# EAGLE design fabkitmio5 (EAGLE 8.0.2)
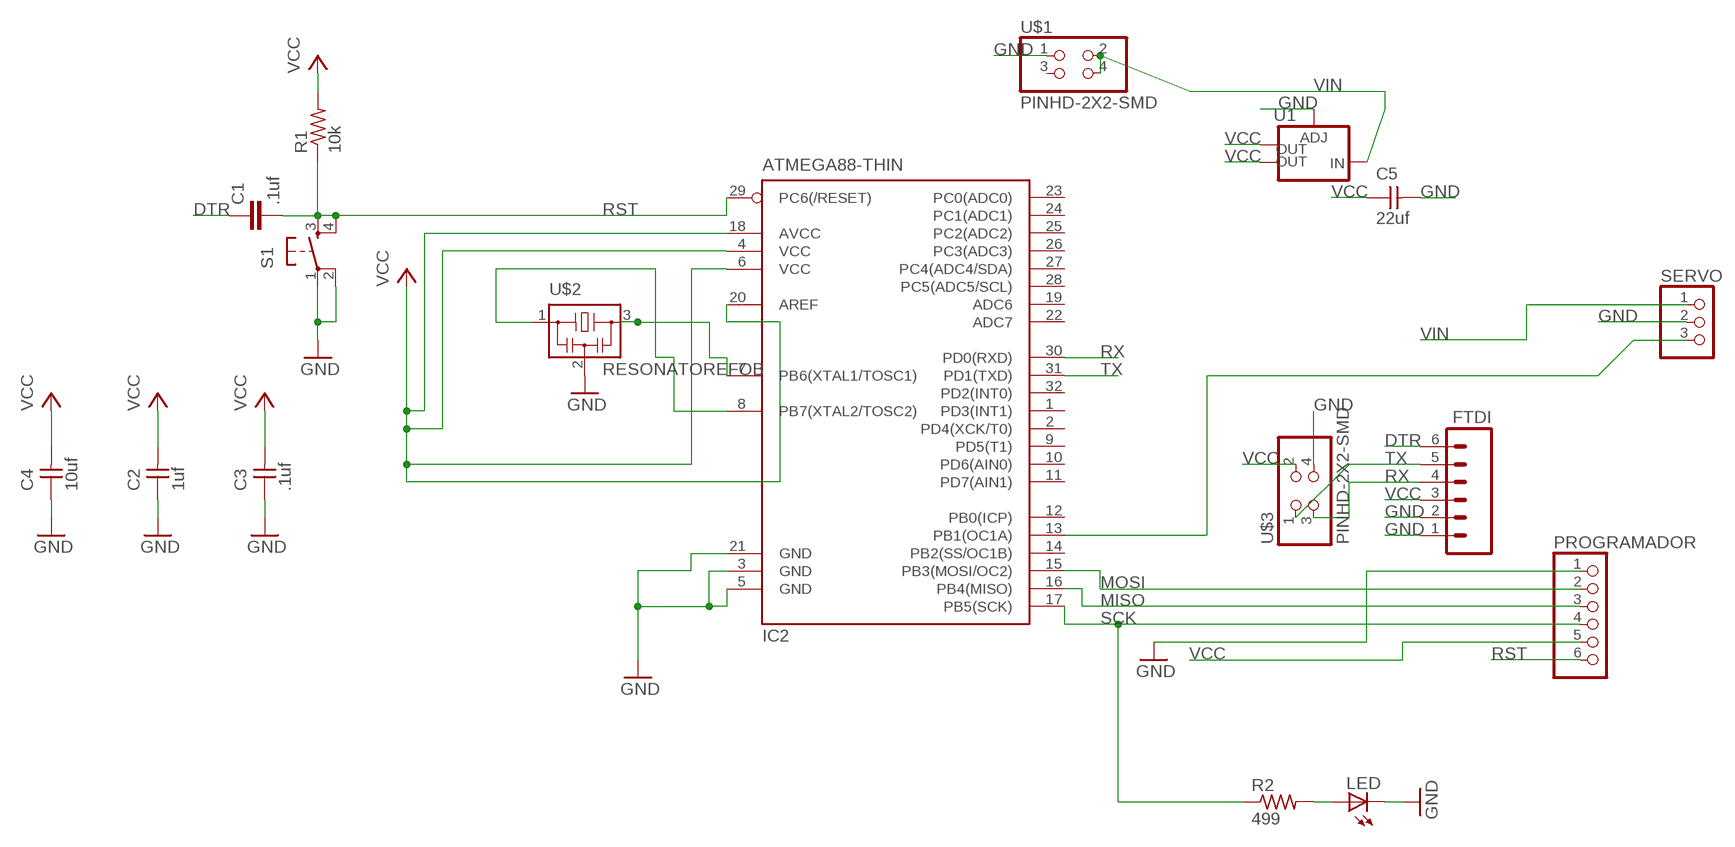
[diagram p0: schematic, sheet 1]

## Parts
C1  .1uf  C-EUC1206  [C1206]
C2  1uf  UNPOLARIZED_CAPACITOR1206  [1206]
C3  .1uf  UNPOLARIZED_CAPACITOR1206  [1206]
C4  10uf  UNPOLARIZED_CAPACITOR1206  [1206]
C5  22uf  CAP-UNPOLARIZEDFAB  [C1206FAB]
FTDI  M06SMD  [1X06-SMD]
IC2  ATMEGA88-THIN  [TQFP32-08THIN]
LED  LED1206  [1206]
PROGRAMADOR  PINHD-1X6  [1X06]
R1  10k  RESISTOR1206  [1206]
R2  499  RESISTOR1206  [1206]
S1  6MM_SWITCH6MM_SWITCH  [6MM_SWITCH]
SERVO  PINHD-1X3  [1X03]
U1  V_REG_LM1117SOT223  [SOT223]
U$1  PINHD-2X2-SMD  [2X02SMD]
U$2  RESONATOREFOB  [EFOBM]
U$3  PINHD-2X2-SMD  [2X02SMD]

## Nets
DTR: C1.1 FTDI.6
GND: C2.1 C3.1 C4.1 C5.2 FTDI.1 FTDI.2 IC2.3(GND) IC2.5(GND) IC2.21(GND) LED.2(C) PROGRAMADOR.1 S1.1(P) S1.2(P1) SERVO.2 U1.1(ADJ) U$1.1 U$2.2 U$3.4
MISO: IC2.16(PB4(MISO)) PROGRAMADOR.3
MOSI: IC2.15(PB3(MOSI/OC2)) PROGRAMADOR.2
N$1: IC2.8(PB7(XTAL2/TOSC2)) U$2.1
N$2: IC2.13(PB1(OC1A)) SERVO.3
N$9: IC2.7(PB6(XTAL1/TOSC1)) U$2.3
N$23: LED.1(A) R2.2
RST: C1.2 IC2.29(PC6(/RESET)) PROGRAMADOR.6 R1.1 S1.3(S) S1.4(S1)
RX: FTDI.4 IC2.30(PD0(RXD)) U$3.3
SCK: IC2.17(PB5(SCK)) PROGRAMADOR.4 R2.1
TX: FTDI.5 IC2.31(PD1(TXD)) U$3.1
VCC: C2.2 C3.2 C4.2 C5.1 FTDI.3 IC2.4(VCC) IC2.6(VCC) IC2.18(AVCC) IC2.20(AREF) PROGRAMADOR.5 R1.2 U1.2(OUT) U1.4(OUT) U$3.2
VIN: SERVO.1 U1.3(IN) U$1.2 U$1.4
Unconnected: IC2.1(PD3(INT1)) IC2.2(PD4(XCK/T0)) IC2.9(PD5(T1)) IC2.10(PD6(AIN0)) IC2.11(PD7(AIN1)) IC2.12(PB0(ICP)) IC2.14(PB2(SS/OC1B)) IC2.19(ADC6) IC2.22(ADC7) IC2.23(PC0(ADC0)) IC2.24(PC1(ADC1)) IC2.25(PC2(ADC2)) IC2.26(PC3(ADC3)) IC2.27(PC4(ADC4/SDA)) IC2.28(PC5(ADC5/SCL)) IC2.32(PD2(INT0)) U$1.3

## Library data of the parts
C1 = rcl:C-EU: CAPACITOR, European symbol
C2-C4 = ng:UNPOLARIZED_CAPACITOR: unpolarized_capacitor
C5 = 01_fab:CAP-UNPOLARIZED
FTDI = SparkFun:M06: Header 6 Standard 6-pin 0.1" header. Use with straight break away headers (SKU : PRT-00116), right angle break away headers (PRT-00553), swiss pins (PRT-00743), machine pins (PRT-00117), and female headers (PRT-00115). Molex polarized connector foot print use with SKU : PRT-08094 with associated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
IC2 = 01_fab:ATMEGA88-THIN
LED = ng:LED
PROGRAMADOR = pinhead:PINHD-1X6: PIN HEADER
R1 R2 = ng:RESISTOR
S1 = ng:6MM_SWITCH: OMRON SWITCH
SERVO = pinhead:PINHD-1X3: PIN HEADER
U1 = 01_fab:V_REG_LM1117: Voltage Regulator LM1117 Standard adjustable voltage regulator but in SMD form. Spark Fun Electronics SKU : COM-00595; PROD_ID: VREG-08170
U$1 U$3 = 01_fab:PINHD-2X2-SMD
U$2 = fab:RESONATOR

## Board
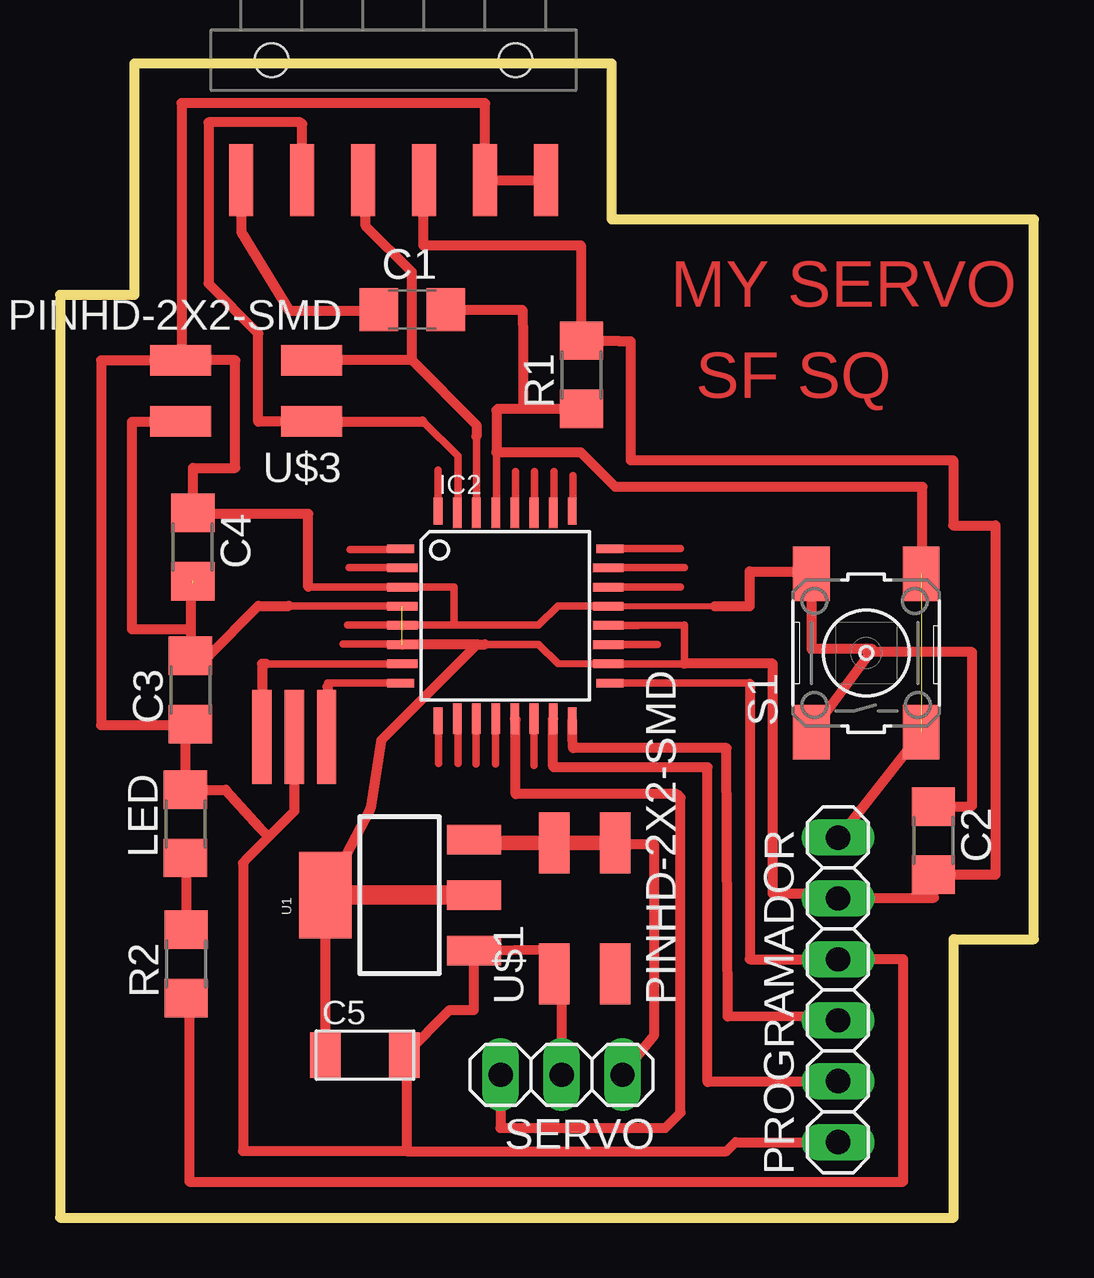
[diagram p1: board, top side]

Size 40.6 x 48.1 mm. Coordinates in mm from the lower left corner, seen from the top.
Outline: 37.25,11.6 37.25,0 0,0 0,38.45 3.1,38.45 3.1,48.1 23,48.1 23,41.6 40.6,41.6 40.6,11.6 37.3,11.6
Copper layers (1*16): Top 0.035mm / dielectric 1.5mm / Bottom 0.035mm
Design rules "default *": minimum track width 15mm, minimum drill 24mil, track to track 0.3985mm, track to pad 0.3985mm, pad to pad 0.3985mm, via to via 0.3985mm, smd to smd 0.3985mm, copper to edge 40mil, drill to drill 8mil, minimum pad ring 10mil, minimum via ring 8mil, stop-mask expansion 4mil, vias tented up to drill 0mil, thermal gap 10mil

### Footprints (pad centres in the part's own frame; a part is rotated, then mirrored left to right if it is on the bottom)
C1206 = smd 1.6 x 1.8: 1 -1.4,0; 2 1.4,0
1206 = smd 1.6 x 1.803: 1 -1.422,0; 2 1.422,0
C1206FAB = smd 1.27 x 1.905: 1 -1.651,0; 2 1.651,0
1X06-SMD = smd 1 x 3: 1 -6.35,5; 2 -3.81,5; 3 -1.27,5; 4 1.27,5; 5 3.81,5; 6 6.35,5 | hole 1.4: -5.08,0; 5.08,0
TQFP32-08THIN = smd 1.118 x 0.356: 1 -4.369,2.8; 8 -4.369,-2.8; 17 4.369,-2.8; 24 4.369,2.8 | smd 1.27 x 0.356: 2 -4.293,2; 3 -4.293,1.2; 4 -4.293,0.4; 5 -4.293,-0.4; 6 -4.293,-1.2; 7 -4.293,-2; 18 4.293,-2; 19 4.293,-1.2; 20 4.293,-0.4; 21 4.293,0.4; 22 4.293,1.2; 23 4.293,2 | smd 0.356 x 1.118: 9 -2.8,-4.369; 16 2.8,-4.369; 25 2.8,4.369; 32 -2.8,4.369 | smd 0.356 x 1.27: 10 -2,-4.293; 14 1.2,-4.293; 15 2,-4.293; 26 2,4.293; 27 1.2,4.293; 31 -2,4.293 | smd 0.35 x 1.27: 11 -1.2,-4.293; 12 -0.4,-4.293; 13 0.4,-4.293; 28 0.4,4.293; 29 -0.4,4.293; 30 -1.2,4.293
1X06 = drill 1.016 long: 1 -6.35,0; 2 -3.81,0; 3 -1.27,0; 4 1.27,0; 5 3.81,0; 6 6.35,0
6MM_SWITCH = smd 2.286 x 1.524: 1 -3.302,2.286; 2 3.302,2.286; 3 -3.302,-2.286; 4 3.302,-2.286
1X03 = drill 1.016 long: 1 -2.54,0; 2 0,0; 3 2.54,0
SOT223 = smd 1.219 x 2.235: 1 -2.311,-3.099; 2 0,-3.099; 3 2.311,-3.099 | smd 3.6 x 2.2: 4 0,3.099
2X02SMD = smd 2.54 x 1.27: 1 -2.54,1.27; 2 2.92,1.27; 3 -2.54,-1.27; 4 2.92,-1.27
EFOBM = smd 0.8 x 3.9: 1 -1.35,0; 2 0,0; 3 1.35,0

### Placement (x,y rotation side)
C1  14.69,37.84 0 top
C2  36.41,15.71 270 top
C3  5.44,21.99 90 top
C4  5.54,27.95 270 top
C5  12.71,6.77 0 top
FTDI  13.91,48.25 180 top
IC2  18.56,25.08 0 top
LED  5.23,16.41 90 top
PROGRAMADOR  32.43,9.49 90 top
R1  21.74,35.13 90 top
R2  5.26,10.57 90 top
S1  33.61,23.53 90 top
SERVO  20.91,5.95 180 top
U1  14.16,13.44 90 top
U$1  21.87,12.69 90 top
U$2  9.77,20.03 180 top
U$3  7.95,34.45 180 top

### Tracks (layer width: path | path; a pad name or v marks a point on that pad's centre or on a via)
DTR
  Top 0.406: FTDI.6 7.56,41.08 9.55,37.81 13.26,37.81 C1.1
GND
  Top 0.254: IC2.21 27.3,25.48 27.31,25.49
  Top 0.305: 10.35,26.29 14.26,26.29 IC2.3 16.42,26.28 16.43,26.29 16.43,24.69 | 16.43,24.69 IC2.5 | 16.43,24.69 19.95,24.69 20.75,25.49 IC2.21
  Top 0.406: IC2.5 | C4.1 5.58,29.81 | C4.1 5.55,29.86 5.55,31.25 7.31,31.25 7.31,35.73 U$3.4 | S1.1 33.77,23.56 | 33.77,23.56 33.87,23.69 31.32,23.69 S1.2 31.32,26.93 28.75,26.93 28.75,25.48 27.3,25.48 | C2.1 37.83,17.13 38.03,17.17 38.03,23.57 33.78,23.57 33.77,23.56 | FTDI.1 FTDI.2 17.72,46.44 17.71,46.45 5.07,46.45 5.07,35.76 U$3.4 | 10.35,26.29 10.35,29.33 5.58,29.33 C4.1 | 8.7,15.87 8.32,16.25 8.32,16.26 6.91,17.83 LED.2 5.23,20.36 C3.1 5.44,20.53 1.71,20.53 1.71,35.72 U$3.4 | 8.7,15.87 7.76,14.93 7.63,14.77 7.63,2.77 14.45,2.77 | U$2.2 9.77,16.94 8.7,15.87 | 14.45,2.77 27.79,2.77 28.16,3.14 PROGRAMADOR.1 | SERVO.2 20.91,9.84 U$1.1 20.53,11.18 U1.1 17.26,8.66 17.25,8.65 16.24,8.65 C5.2 14.45,6.68 14.45,2.77
MISO
  Top 0.406: PROGRAMADOR.3 31.48,8.37 27.84,8.38 27.79,19.57 21.39,19.57 21.36,20.08 IC2.16
MOSI
  Top 0.406: PROGRAMADOR.2 31.6,5.65 26.99,5.65 26.99,18.77 20.59,18.77 20.56,18.8 IC2.15
N$1
  Top 0.305: IC2.8 11.16,22.28 11.15,22.13 | 11.15,19.74 U$2.1
  Top 0.406: 11.15,22.13 11.15,20.06 U$2.1
N$2
  Top 0.406: SERVO.3 18.37,3.75 18.35,3.73 25.23,3.73 25.87,4.37 25.87,17.49 25.71,17.65 18.99,17.65 18.99,20.76 IC2.13
N$9
  Top 0.305: IC2.7 8.59,23.08 8.44,23.08 | U$2.3 8.43,19.72
  Top 0.406: U$2.3 8.42,23.08 8.59,23.08
N$11
  Top 0.305: 18.99,29.17 18.99,31.09
N$12
  Top 0.305: 19.79,29.33 19.79,31.09
N$13
  Top 0.305: 20.59,29.01 20.59,31.09
N$14
  Top 0.305: 21.39,29.17 21.39,30.93
N$15
  Top 0.305: 23.15,27.89 25.87,27.89
N$16
  Top 0.305: 23.15,27.09 26.03,27.09
N$17
  Top 0.305: 22.83,26.29 25.87,26.29
N$18
  Top 0.305: 22.99,23.89 24.91,23.89
N$19
  Top 0.305: 15.79,20.37 15.79,18.93
N$20
  Top 0.305: 16.59,20.53 16.59,18.93
N$21
  Top 0.305: 17.35,20.9 17.35,18.9
N$22
  Top 0.305: 18.15,20.8 18.15,18.9
N$23
  Top 0.406: LED.1 5.26,14.48 R2.2
N$24
  Top 0.305: 19.75,20.7 19.75,18.85
N$25
  Top 0.305: 14.1,23.9 11.8,23.9
N$26
  Top 0.305: 14.3,24.7 12,24.7
N$27
  Top 0.305: 14,27.1 12.05,27.1
N$28
  Top 0.305: 14.05,27.85 12.1,27.85
N$29
  Top 0.305: 15.75,29.5 15.75,31.15
RST  (1 unrouted)
  Top 0.305: 18.19,29.4 IC2.29 18.19,29.4 | 18.19,31.89 18.19,29.4
  Top 0.406: S1.3 32.47,15.84 PROGRAMADOR.6 | R1.1 19.47,33.71 | 19.47,33.71 18.25,33.71 18.19,33.65 18.19,31.89 21.71,31.89 23.15,30.45 35.95,30.45 35.95,26.83 S1.4 | C1.2 19.28,37.84 19.31,36.53 19.31,33.87 19.47,33.71
RX
  Top 0.305: 17.36,32.56 IC2.30
  Top 0.406: 17.36,32.56 17.36,33.04 14.67,35.73 | 14.67,35.73 U$3.3 | 14.67,35.73 14.67,39.41 12.75,41.33 12.75,43.14 FTDI.4
SCK  (1 unrouted)
  Top 0.305: IC2.17 28.74,22.28
  Top 0.406: 5.39,9.65 5.4,9.65 R2.1 5.39,9.15 5.39,1.49 35.15,1.49 35.15,10.77 PROGRAMADOR.4 28.75,10.77 28.75,22.24
TX
  Top 0.305: U$3.1 | 15.11,33.18 15.14,33.18 16.59,31.73 16.59,29.4 IC2.31
  Top 0.406: FTDI.5 10.1,45.58 10.03,45.65 6.19,45.65 6.19,38.93 8.27,36.85 8.27,33.17 U$3.1 | U$3.1 15.11,33.18
VCC  (2 unrouted)
  Top 0.305: 14.26,23.89 IC2.6 | 9.55,25.49 14.26,25.49 IC2.4 | 17.39,23.88 17.71,23.89 19.95,23.89 20.75,23.09 IC2.18 24.9,23.08 | 24.9,23.08 26.03,23.08 26.03,23.09 | 24.9,23.08 26.03,23.09 | IC2.20 24.1,24.68 26.03,24.69 26.03,23.09
  Top 0.406: 5.55,26.45 5.44,26.34 C3.2 | C3.2 5.44,24.53 2.99,24.53 2.99,33.17 U$3.2 | PROGRAMADOR.5 31.81,13.42 | 31.81,13.42 31.44,13.49 29.71,13.49 29.71,23.09 26.03,23.09 | 17.39,23.88 IC2.6 | 17.71,23.89 17.39,23.89 13.39,19.89 12.94,17.06 U1.4 C5.1 | 31.81,13.42 31.9,13.33 36.43,13.33 36.43,14.27 C2.2 38.99,14.29 38.99,28.85 37.23,28.85 37.23,31.57 23.79,31.57 23.79,36.53 23.31,36.53 23.29,36.55 R1.2 21.71,36.58 21.71,40.53 15.15,40.53 15.15,43.22 FTDI.3 | C3.2 6.19,23.41 8.27,25.49 9.55,25.49
  Top 0.813: U1.2 U1.4
VIN
  Top 0.406: SERVO.1 24.75,7.57 24.75,15.57 23.18,15.57 | 23.18,15.57 U$1.4 23.18,15.57
  Top 0.61: U1.3 17.4,15.61 U$1.2 U$1.4

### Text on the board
Top: MY SERVO | SF SQ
